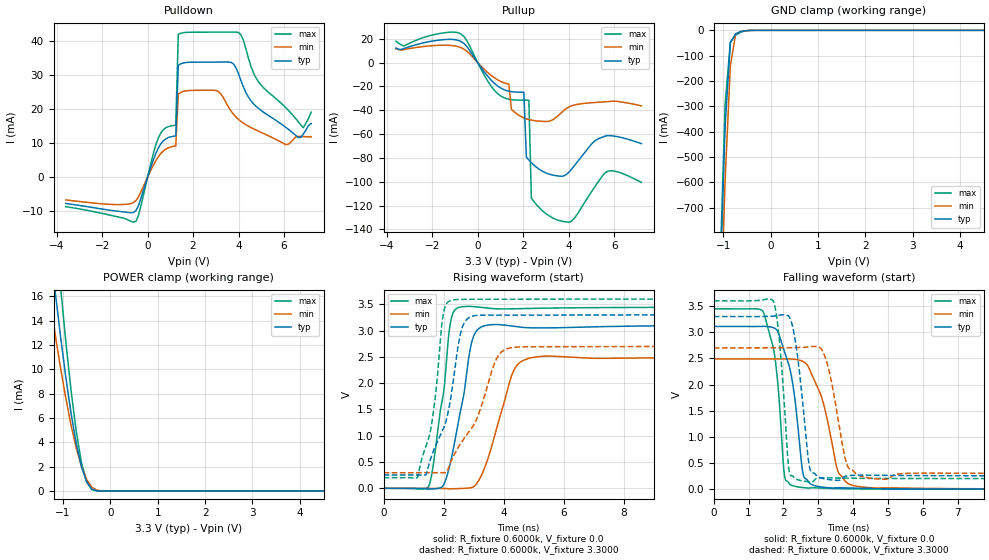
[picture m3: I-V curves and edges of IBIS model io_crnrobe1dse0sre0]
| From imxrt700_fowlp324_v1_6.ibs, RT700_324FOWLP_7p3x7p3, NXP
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[Model] io_crnrobe1dse0sre0
|   Model io_crnrobe1dse0sre0
| This model was characterised for following simulation conditions:
| External (pad) voltage:
|   - Typ: 3.3V,   - Min: 2.7V,   - Max: 3.6V
| Library cells for typ/min/max conditions are connected as defined below:
|  PAD_IO - External Pad
|  ipp_do - Core Input
|  ipp_obe - Output Buffer Enable
|  ASRCN3V3[3] - NC
|  ASRCN3V3[4] - NC
|  ASRCP3V3[4] - NC
|  REFAPBIAS3V3 - gnde
|  REFBAMPL3V3 - vdd1v8
|  REFCAMPH3V3 - vdd1v8
|  REFDNBIAS3V3 - vdd1v8
|  REFH3V3 - REFH3V3
|  REFL3V3 - REFL3V3
|  gnde - gnde
|  ipp_dse - gnde
|  ipp_ina235_3v - NC
|  ipp_ina40_3v - NC
|  ipp_ina_mux - NC
|  ipp_ind - NC
|  ipp_ind_1p8v - NC
|  ipp_ind_3v - NC
|  ipp_sre - gnde
|  vdd - vdd
|  vdd1v8 - vdd1v8
|  vdda - vdde3v3
|  vdde3v3 - vdde3v3
| All other pins connected to ground
Model_type I/O
Polarity   Non-Inverting
Enable   Active-High
Vinl =   0.9900V
Vinh =   2.3100V
Vmeas =  1.6500V
Cref =   15.0000pF
Rref =   0.6000k
Vref =   0.0V
C_comp   4.0038pF   3.8208pF   4.1229pF
|C_comp_pullup   0.5150pF   0.5957pF   0.4948pF
|C_comp_pulldown   2.0816pF   2.1739pF   1.8627pF
[Model Spec]
| variable   typ   min   max
Vinh   2.3100V   NA   NA
Vinl   0.9900V   NA   NA
Vref   0.0V   0.0V   0.0V
Cref   15.0000pF   15.0000pF   15.0000pF
Rref   0.6000k   0.6000k   0.6000k
[Receiver Thresholds]
Vcross_high  =   0.0V
Vcross_low  =   0.0V
Vdiff_ac  =   0.0V
Vdiff_dc  =   0.0V
Tdiffslew_ac  =   0.0S
[Temperature Range]   25.0000   0.1250k   -40.0000
[Voltage Range]   3.3000V   2.7000V   3.6000V
[Pullup Reference]   3.3000V   2.7000V   3.6000V
[Pulldown Reference]   0.0V   0.0V   0.0V
[POWER Clamp Reference]   3.3000V   2.7000V   3.6000V
[GND Clamp Reference]   0.0V   0.0V   0.0V
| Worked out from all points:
|   slope of the pulldown table from 0 to 0.495 V, typ, clamps not added: 56.2 ohm
|   slope of the pullup table from 0 to 0.495 V, typ, clamps not added: 39.2 ohm
|   GND clamp passes 1 mA (typ) near -0.49 V on its own axis
|   POWER clamp passes 1 mA (typ) near -0.52 V on its own axis
|   rising waveform, R_fixture 0.6000k, V_fixture 0.0: 20-80 % time 560ps typ, 747ps min, 427ps max; typ from 0 V to 3.11 V
|   rising waveform, R_fixture 0.6000k, V_fixture 3.3000: 20-80 % time 705ps typ, 1.11ns min, 443ps max; typ from 0.254 V to 3.3 V
|   falling waveform, R_fixture 0.6000k, V_fixture 0.0: 20-80 % time 397ps typ, 553ps min, 284ps max; typ from 3.11 V to 0 V
|   falling waveform, R_fixture 0.6000k, V_fixture 3.3000: 20-80 % time 292ps typ, 388ps min, 223ps max; typ from 3.3 V to 0.254 V
[Pulldown]
|Voltage   I(typ)   I(min)   I(max)
-3.6V     -7.78mA    -6.73mA    -8.72mA
-520mV    -9.932mA   -6.949mA   -13.06mA
470mV     8.52mA     5.95mA     11.49mA
1.24V     12.09mA    9.144mA    15.23mA
1.35V     32.9mA     24.45mA    41.96mA
1.46V     33.31mA    24.89mA    42.28mA
3.11V     33.82mA    25.17mA    42.63mA
3.99V     30.57mA    16.99mA    42.55mA
5.09V     19.13mA    12.85mA    26.34mA
6.08V     14.62mA    9.532mA    20.4mA
6.85V     12.61mA    11.89mA    14.52mA
7.2V      15.74mA    11.8mA     19.11mA
[Pullup]
|Voltage   I(typ)   I(min)   I(max)
-3.6V     12.26mA    11.64mA    18.04mA
-830mV    18.54mA    13.26mA    24.91mA
820mV     -18.75mA   -13.76mA   -24.91mA
1.37V     -23.96mA   -18.01mA   -30.72mA
2.03V     -24.84mA   -46.35mA   -31.51mA
2.14V     -79.26mA   -47.14mA   -31.53mA
2.25V     -81.69mA   -47.75mA   -31.54mA
2.36V     -83.92mA   -48.21mA   -113.8mA
3.24V     -94.07mA   -48.48mA   -129.7mA
4.12V     -89.64mA   -36.31mA   -133.1mA
5.66V     -61.4mA    -32.76mA   -91.66mA
7.2V      -67.96mA   -36.23mA   -100.5mA
[GND_clamp]
|Voltage   I(typ)   I(min)   I(max)
-3.6V     -19.67A    -19.55A    -20.65A
-1.07V    -1.013A    -1.224A    -956.3mA
-960mV    -377.1mA   -587.4mA   -291.7mA
-850mV    -48.2mA    -140.8mA   -46.94mA
-740mV    -13.57mA   -15.62mA   -19.22mA
-630mV    -5.136mA   -4.37mA    -7.235mA
-520mV    -1.276mA   -1.53mA    -1.554mA
-300mV    -4.356uA   -32.48uA   -995.7nA
7.2V      0A         0A         0A
[POWER_clamp]
|Voltage   I(typ)   I(min)   I(max)
-3.6V     102.7mA    81.65mA    131.1mA
-1.38V    23.95mA    18.52mA    31.78mA
-1.27V    20.01mA    15.56mA    26.56mA
-1.16V    16.22mA    12.73mA    21.52mA
-1.05V    12.64mA    10.07mA    16.71mA
-830mV    6.384mA    5.406mA    8.254mA
-720mV    3.9mA      3.518mA    4.888mA
-610mV    1.982mA    2.008mA    2.327mA
-500mV    727.2uA    927.8uA    733.5uA
-390mV    144.5uA    302.5uA    95.96uA
-170mV    198.4nA    4.047uA    20.3nA
7.2V      0A         0A         0A
[Ramp]
| variable   typ   min   max
dV/dt_r  1.8668/0.5597n   1.4948/0.7474n   2.0685/0.4267n
dV/dt_f  1.8274/0.2918n   1.4426/0.3880n   2.0384/0.2227n
R_load = 0.6000k
[Rising Waveform]
R_fixture= 0.6000k
V_fixture= 0.0
V_fixture_min= 0.0
V_fixture_max= 0.0
|time   V(typ)   V(min)   V(max)
0s        139.9nV    3.47uV     132.7nV
1.512ns   -14.1mV    -940.6uV   50.71mV
2.012ns   80.37mV    -1.591mV   1.887V
2.221ns   476.5mV    -9.411mV   3.139V
2.661ns   1.748V     -2.324mV   3.457V
2.91ns    2.72V      11.03mV    3.46V
3.145ns   3.025V     125.4mV    3.449V
4.342ns   3.082V     2.249V     3.415V
5.251ns   3.05V      2.51V      3.426V
60ns      3.111V     2.491V     3.447V
[Rising Waveform]
R_fixture= 0.6000k
V_fixture= 3.3000
V_fixture_min= 2.7000
V_fixture_max= 3.6000
|time   V(typ)   V(min)   V(max)
0s        254.3mV    295.6mV    202.7mV
1.131ns   253.6mV    295.5mV    212.4mV
1.608ns   634.6mV    294.9mV    1.254V
2.011ns   1.159V     295.3mV    3.383V
2.39ns    2.356V     682.5mV    3.589V
2.581ns   2.986V     864.6mV    3.593V
2.811ns   3.234V     1.052V     3.595V
3.779ns   3.295V     2.482V     3.596V
4.456ns   3.295V     2.687V     3.597V
60ns      3.3V       2.7V       3.6V
[Falling Waveform]
R_fixture= 0.6000k
V_fixture= 0.0
V_fixture_min= 0.0
V_fixture_max= 0.0
|time   V(typ)   V(min)   V(max)
0s        3.111V     2.491V     3.447V
1.397ns   3.112V     2.491V     3.411V
1.828ns   3.025V     2.489V     2.088V
2.051ns   2.584V     2.492V     189.9mV
2.25ns    2.081V     2.487V     70.14mV
2.658ns   189.5mV    2.394V     22.93mV
3.134ns   37.31mV    1.671V     18.82mV
3.569ns   27.78mV    329.1mV    9.952mV
4.523ns   12.37mV    26.9mV     3.061mV
60ns      2.412uV    5.566uV    2.123uV
[Falling Waveform]
R_fixture= 0.6000k
V_fixture= 3.3000
V_fixture_min= 2.7000
V_fixture_max= 3.6000
|time   V(typ)   V(min)   V(max)
0s        3.3V       2.7V       3.6V
1.716ns   3.307V     2.7V       3.583V
1.888ns   3.327V     2.699V     2.803V
2.168ns   3.291V     2.702V     331.5mV
2.392ns   2.602V     2.705V     184.2mV
2.752ns   412mV      2.724V     139.8mV
3.239ns   189.2mV    2.439V     216.5mV
3.841ns   256.4mV    437.2mV    209.5mV
4.803ns   263.7mV    190.1mV    204.9mV
60ns      254.3mV    295.6mV    202.7mV
